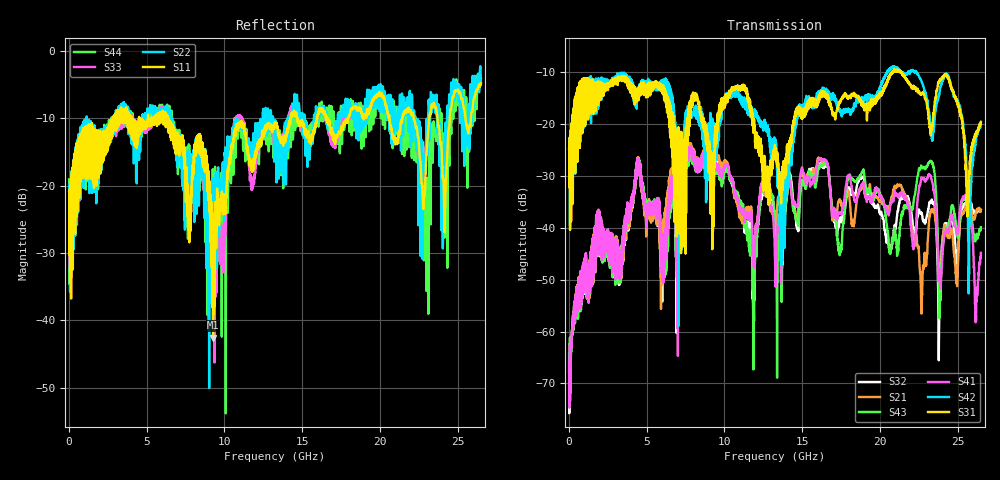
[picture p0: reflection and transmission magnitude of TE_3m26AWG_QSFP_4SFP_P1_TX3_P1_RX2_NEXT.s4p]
!Agilent Technologies,N5222A,MY51421691,A.10.00.00
!Agilent N5222A: A.10.00.00
!Date: Friday, January 30, 2015 12:34:17
!Correction: S11(Full 4 Port(1,2,3,4))
!S12(Full 4 Port(1,2,3,4))
!S13(Full 4 Port(1,2,3,4))
!S14(Full 4 Port(1,2,3,4))
!S21(Full 4 Port(1,2,3,4))
!S22(Full 4 Port(1,2,3,4))
!S23(Full 4 Port(1,2,3,4))
!S24(Full 4 Port(1,2,3,4))
!S31(Full 4 Port(1,2,3,4))
!S32(Full 4 Port(1,2,3,4))
!S33(Full 4 Port(1,2,3,4))
!S34(Full 4 Port(1,2,3,4))
!S41(Full 4 Port(1,2,3,4))
!S42(Full 4 Port(1,2,3,4))
!S43(Full 4 Port(1,2,3,4))
!S44(Full 4 Port(1,2,3,4))
!S4P File: Measurements: <S11,S12,S13,S14>,
!<S21,S22,S23,S24>,
!<S31,S32,S33,S34>,
!<S41,S42,S43,S44>:
# Hz S  dB  R 50.0
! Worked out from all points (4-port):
!   2650 points, 10 MHz to 26.5 GHz, reference 50 ohm
!   strongest paths, dB at 10 MHz, 6.63 GHz, 13.26 GHz, 19.88 GHz, 26.5 GHz:
!     S31: -24.9, -17.8, -24.7, -15.3, -19.6
!     S42: -24.8, -16.2, -25.1, -13.9, -19.8
!     S41: -65.7, -29.6, -46.3, -33.0, -44.8
!     S43: -67.6, -30.7, -38.3, -32.6, -39.9
!     S21: -66.9, -28.6, -39.4, -34.4, -36.5
!     S32: -64.2, -29.6, -37.8, -35.5, -36.6
!   lowest |S11| = -42.5 dB at 9.27 GHz (marker M1), VSWR 1.02, Z = 49.7 + j0.675 ohm
!   |S11| at or under -10 dB: start of sweep to 2.858 GHz; 6.365 GHz to 14.26 GHz (7.893 GHz wide, 76.5 % of centre); 16.62 GHz to 17.98 GHz (1.355 GHz wide, 7.83 % of centre)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
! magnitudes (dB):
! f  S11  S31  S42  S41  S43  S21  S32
! 10 MHz  -20.8  -24.9  -24.8  -65.7  -67.6  -66.9  -64.2
! 4.44 GHz  -10.9  -13.9  -15.0  -29.7  -29.8  -29.6  -29.7
! 9.27 GHz  -42.5  -27.7  -27.6  -27.4  -28.3  -26.0  -26.9
! 10.86 GHz  -11.2  -13.0  -13.8  -34.9  -33.7  -36.0  -34.9
! 13.77 GHz  -13.5  -31.4  -33.6  -37.0  -41.8  -38.4  -43.4
! 16.31 GHz  -8.9  -14.1  -13.7  -26.9  -28.0  -27.5  -28.4
! 26.5 GHz  -4.8  -19.6  -19.8  -44.8  -39.9  -36.5  -36.6
